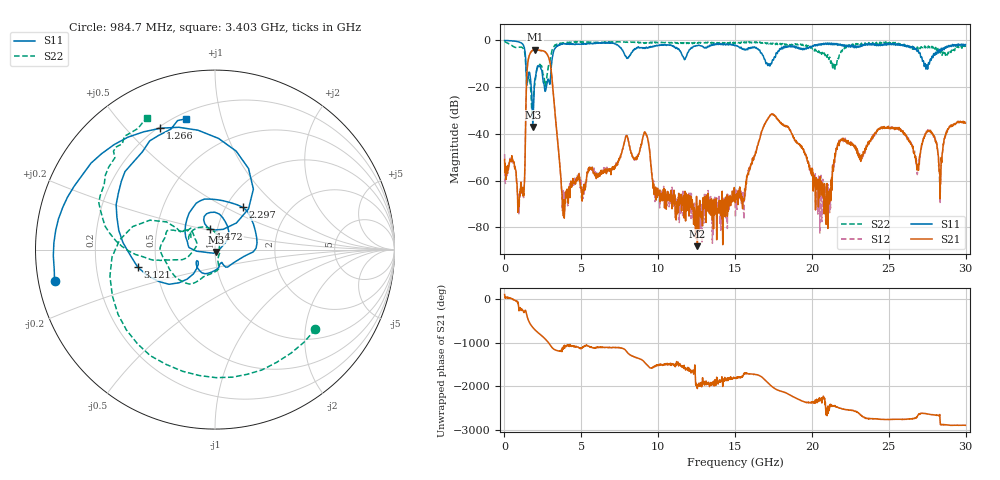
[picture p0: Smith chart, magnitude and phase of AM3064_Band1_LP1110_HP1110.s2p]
# Hz S DB R 50.0
!freq dBS11 angS11 dBS21 angS21 dBS12 angS12 dBS22 angS22
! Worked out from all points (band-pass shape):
!   1600 points, 10 MHz to 29.98 GHz, reference 50 ohm
!   highest |S21| = -3.98 dB at 1.978 GHz (marker M1); lowest = -88.0 dB at 12.55 GHz (marker M2)
!   |S21| within 3 dB of the highest: 1.593 GHz to 2.855 GHz (1.262 GHz wide, 56.8 % of centre)
!   lowest |S11| = -37.0 dB at 1.847 GHz (marker M3), VSWR 1.03, Z = 50.5 - j1.33 ohm
!   |S11| at or under -10 dB: 1.393 GHz to 3.063 GHz (1.671 GHz wide, 75 % of centre); 17.2 GHz to 17.32 GHz (116.7 MHz wide, 0.676 % of centre); 27.36 GHz to 27.57 GHz (206.4 MHz wide, 0.751 % of centre)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
!   |S22| runs from -32.3 to -0.4 dB; largest |S21 - S12| = 0.0085
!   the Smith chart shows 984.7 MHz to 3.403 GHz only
!   S11 on the Smith chart (normalised r, x): 984.7 MHz: 0.05, -0.10; 1.266 GHz: 0.21, +0.63; 1.472 GHz: 0.93, +0.22; 2.297 GHz: 1.20, +0.61; 3.121 GHz: 0.39, -0.10; 3.403 GHz: 0.24, +0.78
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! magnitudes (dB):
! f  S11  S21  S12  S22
! 10 MHz  -0.1  -51.0  -48.6  -0.4
! 984.7 MHz  -0.8  -67.2  -65.3  -2.9
! 1.266 GHz  -2.6  -66.3  -63.1  -4.0
! 1.472 GHz  -18.6  -12.9  -12.9  -15.0
! 1.847 GHz  -37.0  -4.3  -4.2  -28.8
! 1.978 GHz  -16.7  -4.0  -4.0  -18.5
! 2.297 GHz  -11.0  -4.3  -4.3  -10.2
! 3.121 GHz  -7.1  -18.5  -18.3  -3.8
! 3.403 GHz  -2.5  -39.0  -39.2  -1.6
! 3.852 GHz  -1.5  -68.2  -64.8  -1.1
! 5.015 GHz  -1.4  -65.1  -67.5  -0.6
! 9.157 GHz  -3.3  -39.4  -39.1  -1.1
! 10 GHz  -2.2  -66.1  -64.1  -0.9
! 12.55 GHz  -2.3  -88.0  -80.8  -1.2
! 15 GHz  -2.1  -69.2  -66.4  -1.2
! 17.39 GHz  -9.8  -31.5  -31.4  -1.5
! 19.99 GHz  -2.9  -57.2  -58.0  -3.0
! 21 GHz  -1.1  -70.5  -64.2  -6.7
! 21.83 GHz  -1.8  -43.1  -43.0  -6.3
! 25 GHz  -1.3  -37.6  -37.4  -1.1
! 28.35 GHz  -4.8  -61.5  -64.9  -5.4
! 29.98 GHz  -1.8  -35.4  -35.0  -2.9
